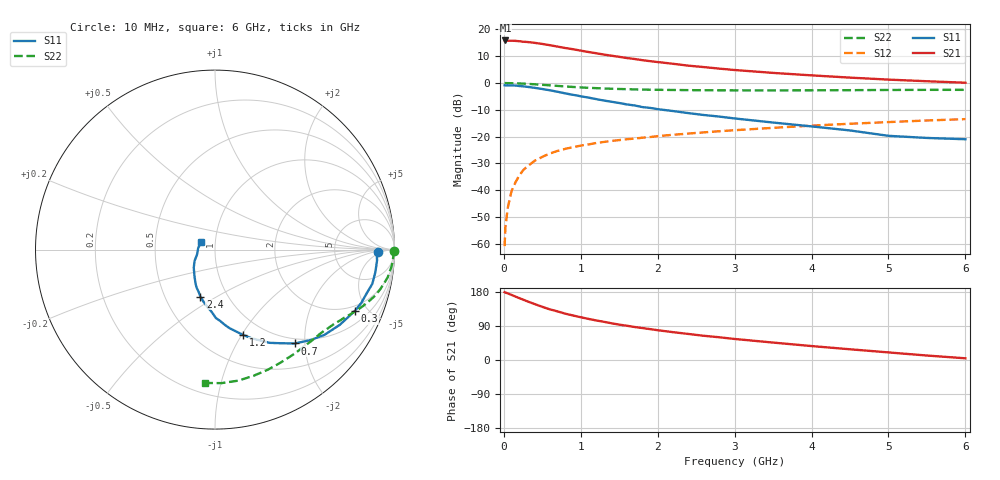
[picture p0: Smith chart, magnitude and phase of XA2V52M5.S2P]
! SIEMENS Discrete & RF Semiconductors
! BFY180
! Si NPN RF Bipolar Junction Transistor in MICRO-X
! VCE = 2.5 V  IC = 2.5 mA
! Common Emitter S-Parameters:  May  1997
# GHz  S  MA  R  50
!  f  S11  S21  S12  S22
! GHz  MAG  ANG  MAG  ANG  MAG  ANG  MAG  ANG
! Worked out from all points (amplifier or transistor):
!   36 points, 10 MHz to 6 GHz, reference 50 ohm
!   highest |S21| = 15.9 dB at 20 MHz (marker M1)
!   |S21| within 3 dB of that: start of sweep to 837.6 MHz
!   unconditionally stable (mu >= 1): 2.289 GHz to end of sweep
!   at 250 MHz: K = 0.16, MSG = 24.0 dB, |S12| = -32.6 dB
!   at 1.4 GHz: K = 0.78, MSG = 15.9 dB, |S12| = -21.6 dB
!   at 6 GHz: K = 1.08, MAG = 5.0 dB, |S12| = -13.5 dB
!   S11 on the Smith chart (normalised r, x): 10 MHz: 21, -3; 300 MHz: 1.67, -4.13; 700 MHz: 0.91, -1.80; 1.2 GHz: 0.80, -1.02; 2.4 GHz: 0.75, -0.42; 6 GHz: 0.85, +0.07
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0.01  0.9086 -0.7  6.148 179.0  0.0009 83.6  0.9953 -0.3
0.02  0.9026 -1.6  6.228 178.1  0.002 90.5  0.9969 -0.7
0.05  0.9048 -3.9  6.162 175.9  0.0046 83.7  0.9945 -1.8
0.1  0.9022 -8.1  6.155 171.8  0.0096 86.2  0.9923 -3.7
0.2  0.8795 -16.1  6.031 163.3  0.0187 80.2  0.9811 -7.2
0.3  0.8507 -23.7  5.84 155.2  0.0273 75.6  0.9655 -10.5
0.4  0.8123 -31.0  5.62 147.6  0.0353 71.5  0.9462 -13.6
0.5  0.7733 -37.9  5.364 140.3  0.0418 68.0  0.9251 -16.4
0.6  0.7305 -43.8  5.073 133.5  0.0484 64.9  0.9029 -18.7
0.7  0.6865 -49.6  4.781 128.2  0.0541 61.6  0.8824 -20.9
0.8  0.6393 -54.7  4.495 122.2  0.0591 59.4  0.8623 -22.9
1.1  0.5337 -67.7  3.791 108.5  0.0714 53.9  0.8138 -27.8
1.2  0.501 -71.7  3.599 104.4  0.0757 52.4  0.8021 -29.4
1.4  0.4467 -79.3  3.232 96.9  0.0829 50.5  0.7813 -32.2
1.7  0.381 -89.3  2.807 87.1  0.0918 47.9  0.7588 -36.2
2.2  0.2996 -102.0  2.284 73.4  0.108 44.5  0.7411 -42.9
2.4  0.2742 -107.2  2.107 68.7  0.1139 43.2  0.7361 -45.4
3  0.218 -119.9  1.749 55.5  0.1315 39.3  0.7293 -53.2
3.5  0.1828 -129.0  1.544 46.0  0.1456 36.1  0.7281 -59.6
4.5  0.1301 -151.0  1.261 28.3  0.1736 28.9  0.7352 -73.0
5.5  0.0943 175.4  1.079 11.8  0.1998 21.3  0.7449 -87.2
6  0.0892 151.3  1.012 4.5  0.2119 17.0  0.7452 -94.4
